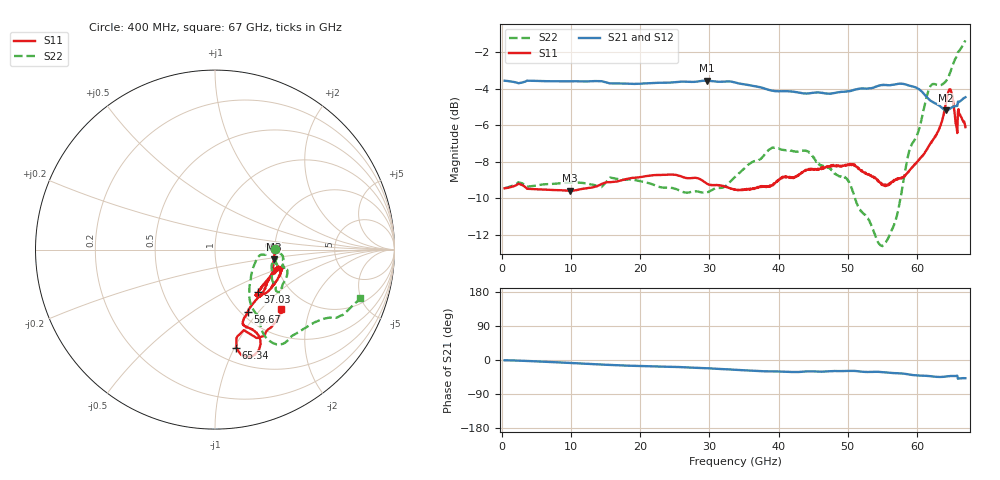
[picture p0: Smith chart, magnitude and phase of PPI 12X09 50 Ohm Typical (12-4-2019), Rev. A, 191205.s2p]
!Keysight Technologies,N5227A,US56070614,A.10.47.06
!Date:	12/4/2019
!Correction
!S11(Full 2 Port(1,2))
!S21(Full 2 Port(1,2))
!S12(Full 2 Port(1,2))
!S22(Full 2 Port(1,2))
!S2P File: Measurements: S11, S21, S12, S22
# GHz S  dB  R 50
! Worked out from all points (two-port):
!   801 points, 400 MHz to 67 GHz, reference 50 ohm
!   highest |S21| = -3.57 dB at 29.62 GHz (marker M1); lowest = -5.2 dB at 64.17 GHz (marker M2)
!   |S21| within 3 dB of the highest: start of sweep to end of sweep
!   lowest |S11| = -9.6 dB at 9.81 GHz (marker M3), VSWR 1.99, Z = 97.7 - j11.4 ohm
!   |S11| at or under -10 dB: nowhere
!   |S22| runs from -12.6 to -1.4 dB; largest |S21 - S12| = 0.0047
!   S11 on the Smith chart (normalised r, x): 400 MHz: 2.01, +0.02; 37.03 GHz: 1.40, -0.75; 59.67 GHz: 1.07, -0.88; 65.34 GHz: 0.64, -1.02; 67 GHz: 1.49, -1.30
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0.4  -9.46 0.9  -3.57 -0.7  -3.55 -0.7  -9.45 1.0
9.81  -9.60 -9.0  -3.60 -7.8  -3.57 -7.8  -9.16 -5.0
11.56  -9.50 -13.3  -3.61 -9.5  -3.59 -9.4  -9.16 -7.7
17.88  -8.97 -22.0  -3.73 -14.7  -3.70 -14.8  -8.99 -13.8
22.63  -8.73 -17.9  -3.69 -17.2  -3.66 -17.2  -9.37 -11.0
29.62  -9.20 -19.4  -3.57 -21.7  -3.53 -21.6  -9.69 -15.9
33.7  -9.55 -34.4  -3.67 -25.9  -3.63 -25.8  -8.85 -28.1
37.03  -9.44 -44.8  -3.90 -29.2  -3.87 -29.2  -7.94 -32.6
42.36  -8.82 -44.4  -4.19 -31.7  -4.16 -31.7  -7.45 -27.7
44.86  -8.43 -32.3  -4.24 -29.9  -4.21 -29.9  -7.69 -15.0
50.68  -8.15 -14.2  -4.10 -28.6  -4.06 -28.7  -9.62 6.0
54.51  -9.09 -21.8  -3.84 -31.4  -3.79 -31.5  -12.50 -14.1
55.93  -9.22 -33.6  -3.82 -33.8  -3.76 -33.9  -12.12 -35.5
59.67  -8.15 -62.2  -3.93 -40.3  -3.88 -40.4  -6.80 -56.8
60.76  -7.72 -66.4  -4.19 -41.4  -4.14 -41.5  -5.53 -60.0
61.84  -7.07 -69.6  -4.62 -42.5  -4.56 -42.6  -3.95 -56.3
64.17  -4.83 -63.9  -5.20 -43.4  -5.13 -43.5  -3.60 -42.5
64.84  -4.05 -72.0  -5.09 -42.3  -5.02 -42.4  -3.09 -34.3
65.34  -5.02 -77.8  -4.97 -42.3  -4.91 -42.5  -2.55 -30.6
65.67  -6.05 -75.5  -4.96 -42.0  -4.89 -42.2  -2.29 -29.6
66.33  -5.53 -51.9  -4.67 -48.2  -4.61 -48.4  -1.82 -25.1
67  -6.11 -41.7  -4.48 -48.0  -4.43 -48.3  -1.37 -18.5
